(* Logix 5000 AddOnInstructionDefinition export Motor_Std; software revision 20.01 *)

TYPE Motor_Std_Type :   // Motor data
STRUCT
   Run_Status : BOOL;   // Run Status (1=running)
   Any_Fail : BOOL;   // Overall Failure Alarm (1= alarm)
   Aux_Fail : BOOL;   // Auxiliary failure alarm (1=alarm)
   OL_Fail : BOOL;   // Overload alarm (1=alarm)
   HOA_Fail : BOOL;   // HOA-switch-not-in-auto alarm (1-alarm)
   Seq_Start : BOOL;   // Motor start initiated from sequence
   Seq_Stop : BOOL;   // Motor stop initiated from sequence
END_STRUCT
END_TYPE

ADD_ON_INSTRUCTION Motor_Std   (* revision 1.3 *)
// Standard motor control
VAR_INPUT
   Aux_Contact : BOOL; {required}   // Auxillary contact physical input
   OL_Trip : BOOL; {required}   // Overload trip contact physical input
   HOA_Switch : BOOL; {required}   // Hand-Off-Auto switch contact physical input (on when in Auto position)
   Alarm_Reset : BOOL; {required}   // Resets alarms
   Maint : BOOL; {required}   // Unit Maintenance/Operate Privilege
   Man_Start : BOOL; {required}   // Manual start for unit
   Man_Stop : BOOL; {required}   // Manual stop for unit
   Select_Dev_Num : DINT; {required}   // Number of device started/stopped at OI
   This_Dev_Num : DINT; {required}   // Number of this device for OI control
END_VAR
VAR_OUTPUT
   Starter : BOOL; {access Read Only, required}   // Motor starter contact physical input
END_VAR
VAR_IN_OUT
   Tag : Motor_Std_Type; {required}   // Motor Tag
END_VAR
VAR
   Start_Req : BOOL;   // Internal used for start logic
   Stop_Req : BOOL;   // Internal used for stop logic
   Fail_Tmr : TIMER := (PRE := 20000);   // Timer for aux-fail alarm
END_VAR

ROUTINE Logic   (* ladder *)
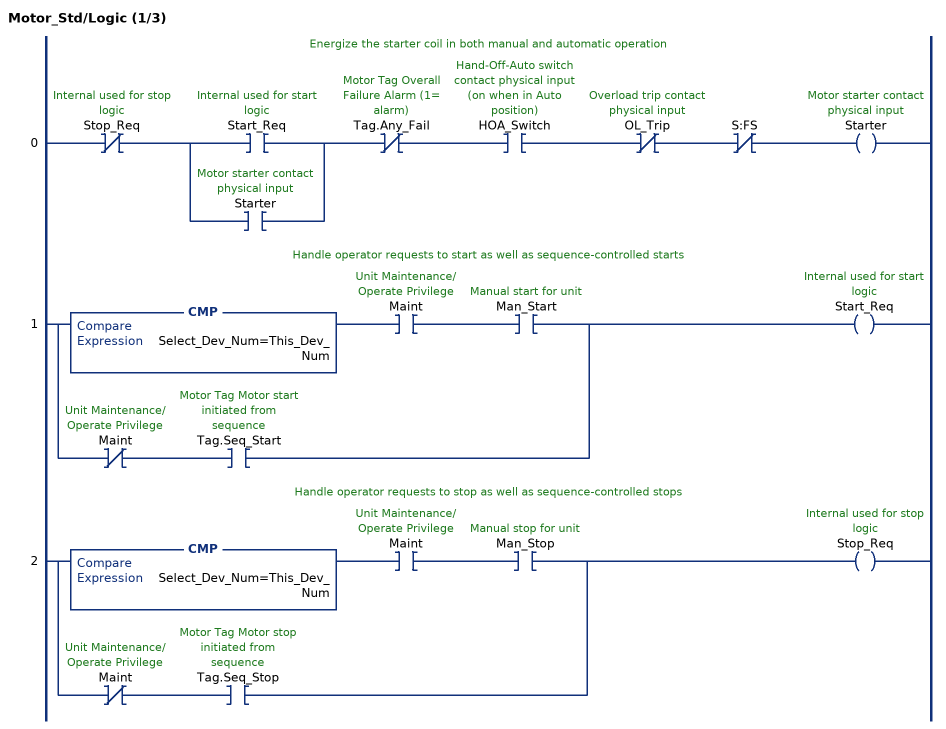
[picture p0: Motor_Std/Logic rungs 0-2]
   // Energize the starter coil in both manual and automatic operation
   0: XIO(Stop_Req)[XIC(Start_Req) ,XIC(Starter) ]XIO(Tag.Any_Fail)XIC(HOA_Switch)XIO(OL_Trip)XIO(S:FS)OTE(Starter);
   // Handle operator requests to start as well as sequence-controlled starts
   1: [CMP(Select_Dev_Num=This_Dev_Num) XIC(Maint) XIC(Man_Start) ,XIO(Maint) XIC(Tag.Seq_Start) ]OTE(Start_Req);
   // Handle operator requests to stop as well as sequence-controlled stops
   2: [CMP(Select_Dev_Num=This_Dev_Num) XIC(Maint) XIC(Man_Stop) ,XIO(Maint) XIC(Tag.Seq_Stop) ]OTE(Stop_Req);
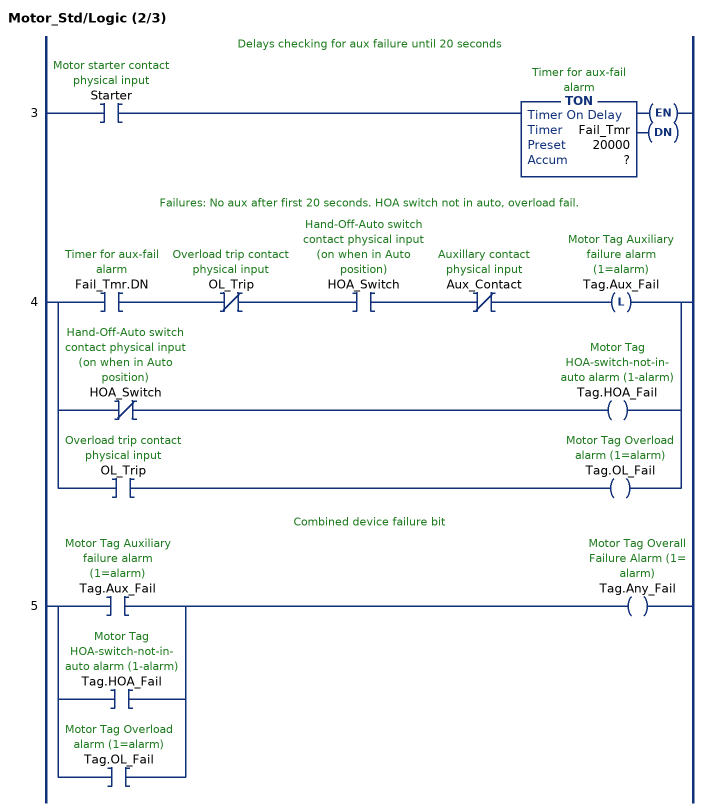
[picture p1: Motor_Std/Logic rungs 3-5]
   // Delays checking for aux failure until 20 seconds
   3: XIC(Starter)TON(Fail_Tmr,?,?);
   // Failures: No aux after first 20 seconds. HOA switch not in auto, overload fail.
   4: [XIC(Fail_Tmr.DN) XIO(OL_Trip) XIC(HOA_Switch) XIO(Aux_Contact) OTL(Tag.Aux_Fail) ,XIO(HOA_Switch) OTE(Tag.HOA_Fail) ,XIC(OL_Trip) OTE(Tag.OL_Fail) ];
   // Combined device failure bit
   5: [XIC(Tag.Aux_Fail) ,XIC(Tag.HOA_Fail) ,XIC(Tag.OL_Fail) ]OTE(Tag.Any_Fail);
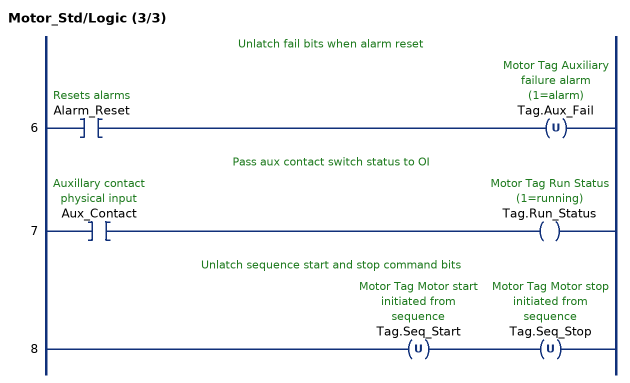
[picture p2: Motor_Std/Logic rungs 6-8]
   // Unlatch fail bits when alarm reset
   6: XIC(Alarm_Reset)OTU(Tag.Aux_Fail);
   // Pass aux contact switch status to OI
   7: XIC(Aux_Contact)OTE(Tag.Run_Status);
   // Unlatch sequence start and stop command bits
   8: OTU(Tag.Seq_Start)OTU(Tag.Seq_Stop);
END_ROUTINE
END_ADD_ON_INSTRUCTION
